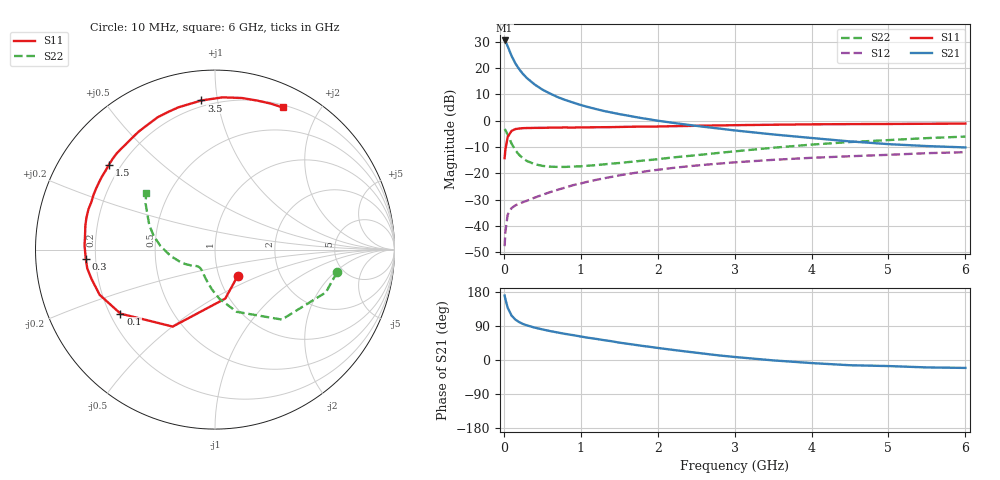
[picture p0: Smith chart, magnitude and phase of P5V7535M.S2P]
! SIEMENS Small Signal Semiconductors
! BFP183
! Si NPN RF Bipolar Junction Transistor in SOT143
! VCE = 0.75 V  IC = 35 mA
! Common Emitter S-Parameters:  March  1996
# GHz  S  MA  R  50
!  f  S11  S21  S12  S22
! GHz  MAG  ANG  MAG  ANG  MAG  ANG  MAG  ANG
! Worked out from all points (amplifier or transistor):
!   36 points, 10 MHz to 6 GHz, reference 50 ohm
!   highest |S21| = 30.5 dB at 10 MHz (marker M1)
!   |S21| within 3 dB of that: start of sweep to 60.84 MHz
!   unconditionally stable (mu >= 1): start of sweep to 20.3 MHz; 215.4 MHz to end of sweep
!   at 250 MHz: K = 1.09, MAG = 22.5 dB, |S12| = -31.0 dB
!   at 1.4 GHz: K = 1.84, MAG = 6.9 dB, |S12| = -21.4 dB
!   at 6 GHz: K = 1.50, MAG = -3.3 dB, |S12| = -12.0 dB
!   S11 on the Smith chart (normalised r, x): 10 MHz: 1.23, -0.37; 100 MHz: 0.24, -0.29; 300 MHz: 0.16, -0.03; 1.5 GHz: 0.15, +0.34; 3.5 GHz: 0.16, +0.90; 6 GHz: 0.23, +1.56
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0.01  0.1932 -48.8  33.4 170.2  0.0041 68.2  0.6917 -10.5
0.02  0.2787 -78.1  32.33 160.8  0.0077 68.8  0.662 -21.1
0.05  0.4894 -118.8  25.89 138.0  0.0163 55.4  0.5391 -46.3
0.1  0.6362 -145.9  17.02 117.3  0.0217 41.1  0.3667 -70.9
0.15  0.6904 -158.6  12.22 106.6  0.0245 38.6  0.2734 -85.1
0.2  0.7065 -166.4  9.459 99.9  0.0264 39.2  0.2223 -94.5
0.25  0.7195 -171.6  7.663 95.0  0.0282 40.4  0.1913 -101.4
0.3  0.7219 -176.0  6.428 91.4  0.03 42.9  0.1707 -107.5
0.4  0.727 178.3  4.866 85.5  0.0343 47.2  0.1487 -116.1
0.5  0.7282 173.9  3.892 80.8  0.0388 48.9  0.1379 -121.7
0.6  0.7345 169.6  3.276 76.4  0.0436 51.3  0.1331 -126.3
0.7  0.7382 165.9  2.794 72.6  0.0484 53.1  0.1317 -130.0
0.8  0.74 162.3  2.462 68.8  0.0534 54.0  0.1318 -132.6
1.1  0.7446 152.8  1.803 58.6  0.0696 55.2  0.1392 -138.9
1.5  0.7571 141.4  1.33 45.9  0.0909 53.2  0.1562 -145.8
1.8  0.7675 132.9  1.11 37.3  0.1059 50.9  0.1732 -150.9
2.2  0.7828 123.0  0.907 26.6  0.1261 46.7  0.1995 -159.0
2.8  0.81 108.8  0.706 12.0  0.1523 39.9  0.2437 -170.5
3.5  0.8344 95.2  0.546 -1.0  0.1795 32.2  0.3047 176.2
4.5  0.8578 80.0  0.402 -13.8  0.2101 21.2  0.3914 159.4
5.5  0.8705 69.2  0.328 -19.6  0.2403 11.6  0.4648 146.3
6  0.877 64.6  0.309 -20.9  0.2509 6.5  0.4966 140.5
